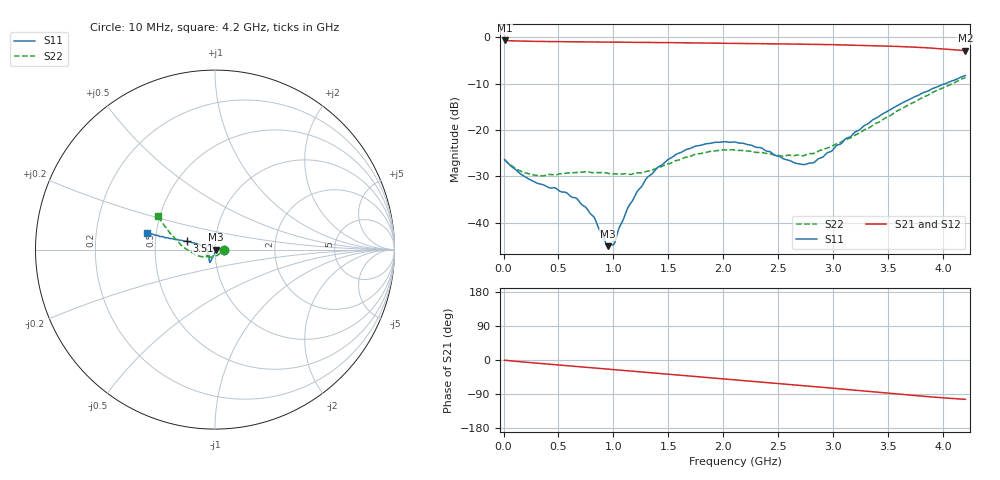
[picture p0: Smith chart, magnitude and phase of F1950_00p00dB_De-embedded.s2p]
! Integrated Device Technology
! Corporate Headquarters
! 6024 Silver Creek Valley Road
! San Jose, CA 95138  USA
! Phone:  1-408-284-8200
! Toll Free:  1-800-223-1366
! Webpage:  http://www.idt.com/
! Timing and RF Division
! 515 Groton Road, Suite 102
! Westford, MA 01886-6024
! Device:  F1950
! Description: 7-bit 0.25 dB Digital Step Attenuator
! Frequency:  150.0 -  4000.00 MHz
! Package:  4x4 mm Thin QFN Plastic Package: 24 pin
! Ports:  2 RF, 12 DC
!  Pin  1  = D0
!  Pin  2  = VDD
!  Pin  3  = Vmode
!  Pin  4  = GND
!  Pin  5  = RF1  =  Port 1
!  Pin  6  = GND
!  Pin  7  = GND
!  Pin  8  = GND
!  Pin  9  = GND
!  Pin 10  = GND
!  Pin 11  = GND
!  Pin 12  = GND
!  Pin 13  = GND
!  Pin 14  = RF2  =  Port 2
!  Pin 15  = GND
!  Pin 16  = LE
!  Pin 17  = CLK
!  Pin 18  = DATE
!  Pin 19  = D6
!  Pin 20  = D5
!  Pin 21  = D4
!  Pin 22  = D3
!  Pin 23  = D2
!  Pin 24  = D1
! State:  0
! Atten State:  0.00 dB
! Voltage:  +5.00 Volts
! Current:  Not Measured mA
! Data:  The device was measured on a the F195X evaluation board which has
!  individual transmission lines to the RF pins.  Data was collected
!  using a calibrated network analyzer.  The evaluation board was
!  de-embedded using a TRL calibration technique.
!  The reference plane is the edge of the package pin.
! Misc:  Board 2019
!  Action Tracker AT0250
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# GHz S dB R 50
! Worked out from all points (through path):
!   420 points, 10 MHz to 4.2 GHz, reference 50 ohm
!   highest |S21| = -0.65 dB at 10 MHz (marker M1); lowest = -2.9 dB at 4.2 GHz (marker M2)
!   group delay of S21, straight-line fit = 68.8 ps
!   lowest |S11| = -45.0 dB at 950 MHz (marker M3), VSWR 1.01, Z = 50.5 - j0.122 ohm
!   |S11| at or under -10 dB: start of sweep to 4.014 GHz
!   |S22| runs from -29.9 to -8.7 dB; largest |S21 - S12| = 0.0011
!   S11 on the Smith chart (normalised r, x): 10 MHz: 1.10, -0.00; 3.51 GHz: 0.72, +0.07; 4.2 GHz: 0.45, +0.10
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0.01  -26.35 -2.3  -0.65 -0.6  -0.65 -0.6  -26.31 -3.5
0.14  -29.16 -5.8  -0.78 -4.2  -0.78 -4.2  -28.68 -7.1
0.29  -31.28 8.4  -0.85 -8.0  -0.85 -8.0  -29.74 -1.4
0.57  -33.48 31.0  -0.93 -14.8  -0.92 -14.8  -29.27 0.9
0.71  -36.03 33.9  -0.95 -18.2  -0.95 -18.2  -29.08 -7.6
0.82  -38.69 28.4  -0.97 -20.9  -0.97 -20.9  -29.19 -15.4
0.95  -45.03 -12.5  -1.00 -24.1  -1.00 -24.1  -29.29 -29.5
1.01  -44.39 -53.2  -1.01 -25.5  -1.01 -25.6  -29.41 -37.0
1.13  -36.80 -92.3  -1.04 -28.5  -1.04 -28.5  -29.46 -55.1
1.22  -33.11 -100.3  -1.06 -30.7  -1.05 -30.7  -29.21 -69.0
1.31  -30.13 -104.3  -1.07 -32.9  -1.07 -32.9  -28.81 -84.0
1.41  -27.91 -106.3  -1.10 -35.3  -1.10 -35.3  -28.09 -98.0
1.57  -25.22 -108.7  -1.14 -39.2  -1.14 -39.2  -26.57 -116.6
1.74  -23.49 -110.3  -1.18 -43.4  -1.18 -43.4  -25.23 -130.4
2.11  -22.59 -114.1  -1.29 -52.5  -1.29 -52.5  -24.31 -145.9
2.34  -23.79 -120.7  -1.35 -58.1  -1.35 -58.1  -24.81 -147.1
2.66  -27.16 -148.1  -1.44 -66.0  -1.44 -66.0  -25.41 -140.0
2.81  -27.08 -170.0  -1.49 -69.8  -1.49 -69.8  -25.06 -138.6
3.15  -21.50 163.6  -1.64 -78.5  -1.63 -78.5  -21.72 -151.5
3.51  -15.67 163.6  -1.88 -87.9  -1.87 -87.9  -16.96 -176.3
3.81  -11.98 165.8  -2.19 -95.4  -2.19 -95.5  -12.97 166.0
4.2  -8.22 165.8  -2.87 -103.8  -2.87 -103.9  -8.67 149.5
